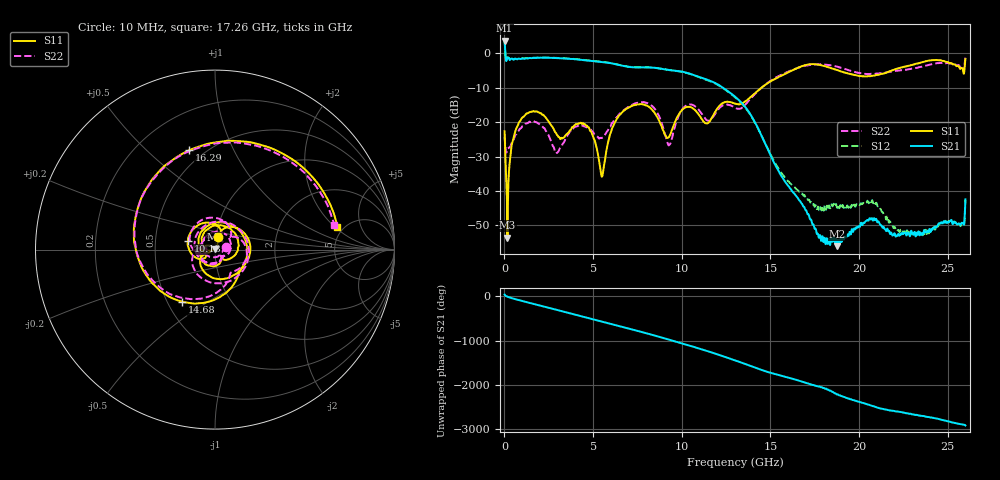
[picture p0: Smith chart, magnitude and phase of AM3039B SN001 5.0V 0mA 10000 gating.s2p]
!Agilent Technologies,E8364B,MY43040894,A.07.50.67
!Agilent E8364B: A.07.50.67
!Date: Tuesday, June 28, 2016 08:07:15
!Correction: S11(Full 2 Port(1,2))
!S21(Full 2 Port(1,2))
!S12(Full 2 Port(1,2))
!S22(Full 2 Port(1,2))
!S2P File: Measurements: S11, S21, S12, S22:
# Hz S  dB  R 50
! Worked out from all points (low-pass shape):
!   1601 points, 10 MHz to 26 GHz, reference 50 ohm
!   highest |S21| = 3.66 dB at 10 MHz (marker M1); lowest = -56.1 dB at 18.77 GHz (marker M2)
!   |S21| within 3 dB of the highest: start of sweep to 44.32 MHz
!   lowest |S11| = -53.6 dB at 172.4 MHz (marker M3), VSWR 1.00, Z = 49.8 + j0.125 ohm
!   |S11| at or under -10 dB: start of sweep to 14.5 GHz
!   |S22| runs from -29.0 to -0.9 dB; largest |S21 - S12| = 0.027
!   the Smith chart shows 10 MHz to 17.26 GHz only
!   S11 on the Smith chart (normalised r, x): 10 MHz: 1.02, +0.15; 10.13 GHz: 0.73, +0.07; 14.68 GHz: 0.60, -0.39; 16.29 GHz: 0.42, +0.69; 17.26 GHz: 4.41, +2.17
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1e7  -22.67 78.2  3.66 40.7  3.73 41.6  -24.27 15.8
1.724375e8  -53.55 143.2  -1.25 -8.5  -1.19 -8.3  -27.75 -60.8
8.871625e8  -19.69 131.2  -1.63 -93.1  -1.58 -93.0  -21.87 149.2
1.666862e9  -16.86 50.2  -1.35 -173.8  -1.31 -173.6  -19.72 51.9
2.690219e9  -21.21 -40.8  -1.35 81.0  -1.28 81.2  -26.39 -46.1
3.502406e9  -23.53 -57.4  -1.56 -2.6  -1.50 -2.4  -24.44 -55.1
4.347081e9  -20.37 -126.8  -1.92 -90.5  -1.88 -90.4  -21.03 -153.1
5.938969e9  -23.84 -168.7  -2.83 101.8  -2.79 102.0  -21.40 -121.5
6.962325e9  -15.91 66.6  -3.91 -5.3  -3.89 -4.8  -15.70 68.3
8.684162e9  -19.20 -138.8  -4.37 169.3  -4.36 169.9  -17.91 -165.2
1.012986e10  -16.00 162.2  -5.47 3.0  -5.51 3.4  -15.71 146.1
1.152682e10  -20.10 72.2  -7.86 -168.4  -7.96 -168.3  -19.64 39.4
1.3005e10  -14.64 -26.0  -12.61 -7.2  -12.80 -7.9  -15.81 -47.6
1.467811e10  -9.30 -122.1  -25.94 110.7  -25.84 104.9  -9.22 -132.9
1.628624e10  -4.85 104.5  -40.43 -68.1  -38.62 -91.4  -4.76 96.8
1.726086e10  -3.18 10.6  -48.29 172.1  -43.37 139.0  -3.36 11.6
1.734208e10  -3.15 2.4  -49.19 159.0  -43.61 126.5  -3.32 4.4
1.877153e10  -4.86 -131.9  -56.06 -57.6  -44.94 -60.4  -3.88 -121.1
2.167916e10  -5.31 18.9  -51.64 -54.8  -49.21 -68.0  -5.47 26.4
2.317359e10  -3.08 -93.1  -52.78 -165.0  -52.07 -163.0  -4.30 -82.2
2.427816e10  -1.97 177.2  -50.44 123.3  -51.26 119.5  -3.00 -166.1
2.6e10  -1.70 -18.1  -42.46 -40.7  -42.61 -40.1  -0.92 13.7
